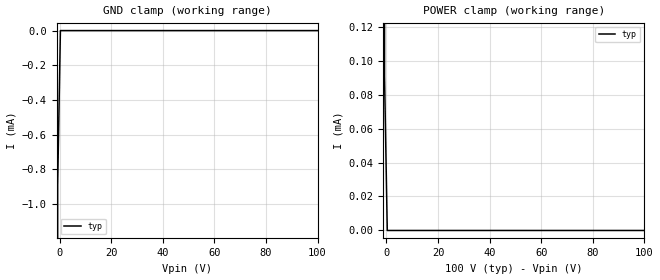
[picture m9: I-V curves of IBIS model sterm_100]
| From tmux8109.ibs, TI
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| sterm_100
[Model]   sterm_100
Model_type   Terminator
|   typ   min   max
C_comp   4.014581e-12   NA   NA
[Voltage Range]   100   NA   NA
[Temperature Range]   27   NA   NA
[Power Clamp Reference]   100   NA   NA
[GND Clamp Reference]   0   NA   NA
[GND Clamp]
|   Voltage   I(typ)   I(min)   I(max)
-5V       -1.133A    NA         NA
-1.818V   -181.5mA   NA         NA
-757.6mV  -886.5uA   NA         NA
303mV     -653.1pA   NA         NA
100V      3.296nA    NA         NA
[POWER Clamp]
|   Voltage   I(typ)   I(min)   I(max)
-5V       744mA      NA         NA
-1.818V   145.4mA    NA         NA
-758mV    90.5uA     NA         NA
303mV     3.293nA    NA         NA
100V      -690.1pA   NA         NA
